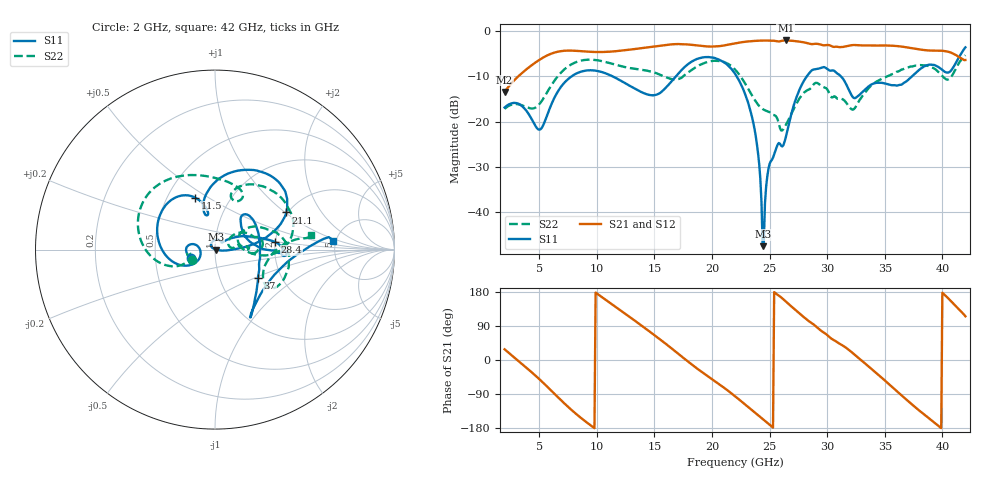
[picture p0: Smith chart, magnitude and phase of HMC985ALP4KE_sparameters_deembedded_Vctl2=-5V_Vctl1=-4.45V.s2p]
!s2p File: Measurements: S11, S21, S12, S22
# GHz S dB R 50.0
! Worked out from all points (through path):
!   401 points, 2 GHz to 42 GHz, reference 50 ohm
!   highest |S21| = -2.06 dB at 26.4 GHz (marker M1); lowest = -13.4 dB at 2 GHz (marker M2)
!   lowest |S11| = -47.5 dB at 24.4 GHz (marker M3), VSWR 1.01, Z = 50.4 + j0.0139 ohm
!   |S11| at or under -10 dB: start of sweep to 7.806 GHz; 22.15 GHz to 28.23 GHz (6.084 GHz wide, 24.2 % of centre); 31.2 GHz to 37.36 GHz (6.163 GHz wide, 18 % of centre)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
!   |S22| runs from -21.9 to -5.3 dB; largest |S21 - S12| = 0.00094
!   S11 on the Smith chart (normalised r, x): 2 GHz: 0.76, -0.07; 11.5 GHz: 0.68, +0.44; 21.1 GHz: 1.97, +1.02; 28.4 GHz: 2.00, +0.19; 37 GHz: 1.52, -0.52; 42 GHz: 4.76, +0.84
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2  -16.86 -161.7  -13.43 28.2  -13.44 28.2  -17.17 -155.6
5  -21.76 -172.5  -6.38 -50.1  -6.38 -50.1  -16.18 -159.8
6.3  -14.83 -150.4  -4.76 -88.3  -4.76 -88.3  -11.04 -161.6
8.7  -8.90 150.3  -4.44 -154.6  -4.44 -154.5  -6.47 151.3
11.5  -10.15 111.1  -4.47 143.2  -4.47 143.2  -7.33 105.2
13.6  -13.11 101.1  -3.85 97.2  -3.85 97.2  -8.43 75.8
15.4  -13.81 105.8  -3.25 56.5  -3.25 56.5  -9.52 62.3
17.9  -7.33 80.2  -2.95 -3.5  -2.94 -3.5  -9.17 72.2
21.1  -6.98 27.5  -3.14 -74.4  -3.14 -74.3  -6.87 16.1
22  -9.39 16.9  -2.71 -95.6  -2.71 -95.5  -8.47 0.7
23.6  -20.40 -0.2  -2.18 -135.3  -2.18 -135.2  -14.73 -3.9
24  -26.96 -7.2  -2.11 -145.3  -2.11 -145.3  -16.22 1.6
24.4  -47.49 1.9  -2.08 -155.4  -2.08 -155.4  -17.20 7.3
25  -29.34 133.3  -2.11 -170.7  -2.11 -170.6  -17.90 11.0
26.4  -23.52 42.6  -2.06 154.6  -2.06 154.7  -20.77 33.1
28.4  -9.42 7.2  -2.73 102.7  -2.73 102.7  -12.91 18.5
28.7  -8.60 2.1  -2.87 96.5  -2.87 96.5  -12.20 16.6
32.5  -14.69 32.9  -3.08 10.8  -3.08 10.8  -16.62 28.5
35.4  -11.79 19.1  -3.19 -64.6  -3.19 -64.6  -9.80 19.5
37  -10.83 -33.4  -3.61 -107.7  -3.61 -107.7  -8.02 5.2
39.8  -8.17 -56.9  -4.33 -177.2  -4.32 -177.1  -9.35 -35.0
42  -3.59 4.3  -6.38 115.2  -6.39 115.3  -5.33 8.9
